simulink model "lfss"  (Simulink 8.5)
settings: Solver=ode45  StartTime=0.0  StopTime=40  RelTol=1e-3
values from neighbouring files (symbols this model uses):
  Ave = [    [vehicle_flex34.m]    (also in vehicle_rigid.m)
  Bve = [    [vehicle_flex34.m]    (also in vehicle_rigid.m)
  Cve = [    [vehicle_flex34.m]    (also in vehicle_rigid.m)
  Dve = [    [vehicle_flex34.m]    (also in vehicle_rigid.m)

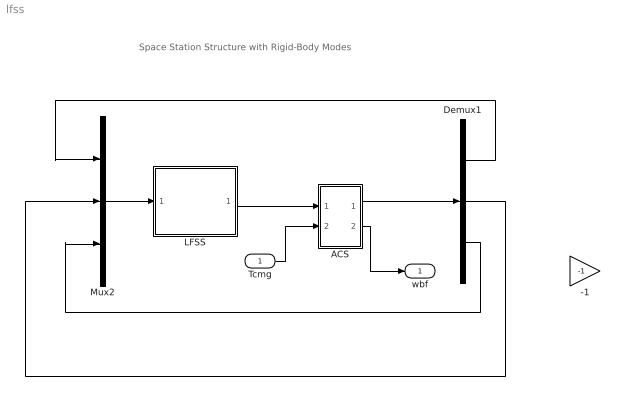
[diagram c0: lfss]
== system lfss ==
  note: Space Station Structure with Rigid-Body Modes
  Tcmg : Inport
  -1 : Gain  Gain=-1
  ACS : Subsystem
  Demux1 : Demux  Outputs=3
  LFSS : Subsystem
  Mux2 : Mux  Inputs=3
  wbf : Outport
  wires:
  Mux2/1 -> LFSS/1(Tcmg)
  Demux1/2 -> Mux2/2
  Demux1/1 -> Mux2/1
  ACS/1(Tq) -> Demux1/1
  LFSS/1(wbf) -> ACS/1(wb)
  Demux1/3 -> Mux2/3
  Tcmg/1 -> ACS/2(atc)
  ACS/2(the) -> wbf/1

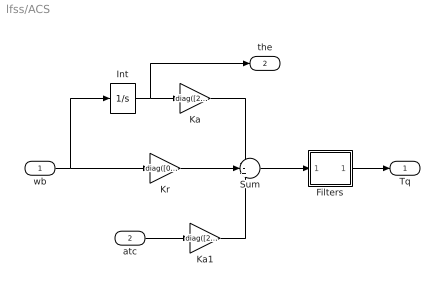
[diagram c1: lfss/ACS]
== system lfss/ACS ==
  wb : Inport
  atc : Inport  Port=2
  Filters : Subsystem
  Int : Integrator
  Ka : Gain  Gain=diag([275000, 80000, 250000])  Multiplication=Matrix(K*u)
  Ka1 : Gain  Gain=diag([275000, 80000, 250000])  Multiplication=Matrix(K*u)
  Kr : Gain  Gain=diag([0.77e7, 0.224e7, 0.7e7])  Multiplication=Matrix(K*u)
  Sum : Sum  Inputs=--+
  Tq : Outport
  the : Outport  Port=2
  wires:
  wb/1 -> Int/1, Kr/1
  Sum/1 -> Filters/1(I)
  Kr/1 -> Sum/2
  Int/1 -> Ka/1, the/1
  Ka/1 -> Sum/1
  Filters/1(O) -> Tq/1
  atc/1 -> Ka1/1
  Ka1/1 -> Sum/3

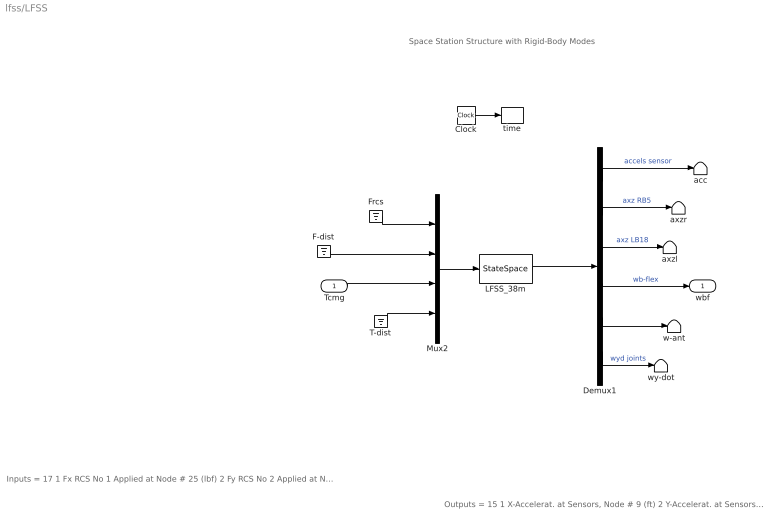
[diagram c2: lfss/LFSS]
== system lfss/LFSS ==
  note: Space Station Structure with Rigid-Body Modes
  note: Inputs = 17 1 Fx RCS No 1 Applied at Node # 25 (lbf) 2 Fy RCS No 2 Applied at Node # 25 (lbf) 3 Fx RCS No 3 Applied at Node # 26 (lbf) 4 Fy RCS No 4 Applied at Node # 26 (lbf) 5 Fx RCS No 5 Applied at Node # 27 (lbf) 6 Fy RCS No 6 Applied at Node # 27 (lbf) 7 Fx RCS No 7 Applied at Node # 28 (lbf) 8 Fy RCS No 8 Applied at Node # 28 (lbf) 9 Fx Disturb. No 9 at Node # 21 (lbf) 10 Fy Disturb. No 10 at Node # 21 (lbf) 11 Fz Disturb. No 11 at Node # 21 (lbf) 12 Torq-x No 1 CMG Applied at Node # 10 (ft-lb) 13 Torq-y No 2 CMG Applied at Node # 10 (ft-lb) 14 Torq-z No 3 CMG Applied at Node # 10 (ft-lb) 15 Torq-x No 4 Gimbal Dist. at Node # 1 (ft-lb) 16 Torq-y No 5 Gimbal Dist. at Node # 1 (ft-lb) 17 Torq-z No 6 Gimbal Dist. at Node # 1 (ft-lb)
  note: Outputs = 15 1 X-Accelerat. at Sensors, Node # 9 (ft) 2 Y-Accelerat. at Sensors, Node # 9 (ft) 3 Z-Accelerat. at Sensors, Node # 9 (ft) 4 X-Accelerat. at Right Boom End, Node # 5 (ft) 5 Z-Accelerat. at Right Boom End, Node # 5 (ft) 6 X-Accelerat. at Left Boom End, Node # 18 (ft) 7 Z-Accelerat. at Left Boom End, Node # 18 (ft) 8 X-Rot. Rate at Sensors, Node # 9 (radian) 9 Y-Rot. Rate at Sensors, Node # 9 (radian) 10 Z-Rot. Rate at Sensors, Node # 9 (radian) 11 X-Rot. Rate at Antena Bot-Left, Node # 24 (radian) 12 Y-Rot. Rate at Antena Bot-Left, Node # 24 (radian) 13 Z-Rot. Rate at Antena Bot-Left, Node # 24 (radian) 14 Y-Rot.Accel. at Right Joint, Node # 7 (radian) 15 Y-Rot.Accel. at Left Joint, Node # 16 (radian)
  Tcmg : Inport
  Clock : Clock
  Demux1 : Demux  Outputs=[3, 2, 2, 3, 3, 2]
  F-dist : Ground
  Frcs : Ground
  LFSS_38m : StateSpace  A=Ave  B=Bve  C=Cve  D=Dve  X0=0
  Mux2 : Mux  Inputs=[8, 3, 3, 3]
  T-dist : Ground
  acc : Terminator
  axzl : Terminator
  axzr : Terminator
  time : ToWorkspace  VariableName=time  SampleTime=-1
  w-ant : Terminator
  wy-dot : Terminator
  wbf : Outport
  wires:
  Mux2/1 -> LFSS_38m/1
  Clock/1 -> time/1
  LFSS_38m/1 -> Demux1/1
  Demux1/1 -> acc/1  "accels sensor"
  Demux1/4 -> wbf/1  "wb-flex"
  Tcmg/1 -> Mux2/3
  Demux1/2 -> axzr/1  "axz RB5"
  Frcs/1 -> Mux2/1
  Demux1/3 -> axzl/1  "axz LB18"
  F-dist/1 -> Mux2/2
  T-dist/1 -> Mux2/4
  Demux1/5 -> w-ant/1
  Demux1/6 -> wy-dot/1  "wyd joints"

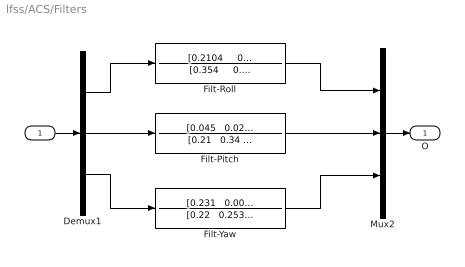
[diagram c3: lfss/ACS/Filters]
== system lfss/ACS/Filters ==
  I : Inport
  Demux1 : Demux  Outputs=3
  Filt-Pitch : TransferFcn  Numerator="[0.045   0.025   1]"  Denominator="[0.21   0.34     1]"
  Filt-Roll : TransferFcn  Numerator="[0.2104     0.036  1]"  Denominator="[0.354     0.131    1]"
  Filt-Yaw : TransferFcn  Numerator="[0.231   0.0025  1]"  Denominator="[0.22   0.253   1]"
  Mux2 : Mux  Inputs=3
  O : Outport
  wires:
  Filt-Yaw/1 -> Mux2/3
  Filt-Pitch/1 -> Mux2/2
  Filt-Roll/1 -> Mux2/1
  Demux1/2 -> Filt-Pitch/1
  Demux1/1 -> Filt-Roll/1
  Demux1/3 -> Filt-Yaw/1
  I/1 -> Demux1/1
  Mux2/1 -> O/1
